FUNCTION_BLOCK FB_CylinderTempRecord EXTENDS FB_CylinderTemp
VAR_INPUT
	bRecordStart		: BOOL;
	tIntervalTime		: TIME;
END_VAR
VAR_OUTPUT
	bRecordDone			: BOOL;
	aTemps				: ARRAY[1..100] OF LREAL;
END_VAR
VAR
	fbTimerInterval		: TON;
	nIndex				: INT;
END_VAR

// =========================================================
;
// =========================================================

METHOD PUBLIC M_Record
VAR_INPUT
END_VAR
// =========================================================
	// Recording array filled
	
bRecordDone := (nIndex = 100);

// =========================================================
	// Recording temperatures
	
IF bRecordStart AND NOT bRecordDone AND NOT fbTimerInterval.Q THEN
	fbTimerInterval( IN := TRUE, PT := tIntervalTime );
END_IF

IF fbTimerInterval.Q THEN
	fbTimerInterval( IN := FALSE );
	nIndex := nIndex + 1;
	aTemps[nIndex] := lrTempCurrent;
END_IF

// =========================================================
END_METHOD

METHOD PUBLIC M_Reset
VAR_INPUT
END_VAR
// =========================================================
	// Reset
	
SUPER^.M_Reset();					// Calling method M_Reset of base class FB_Cylinder via 'SUPER^.'

FOR nIndex := 1 TO 100 BY 1 DO
	aTemps[nIndex] := 0;
END_FOR

nIndex := 0;

// =========================================================
END_METHOD

END_FUNCTION_BLOCK
